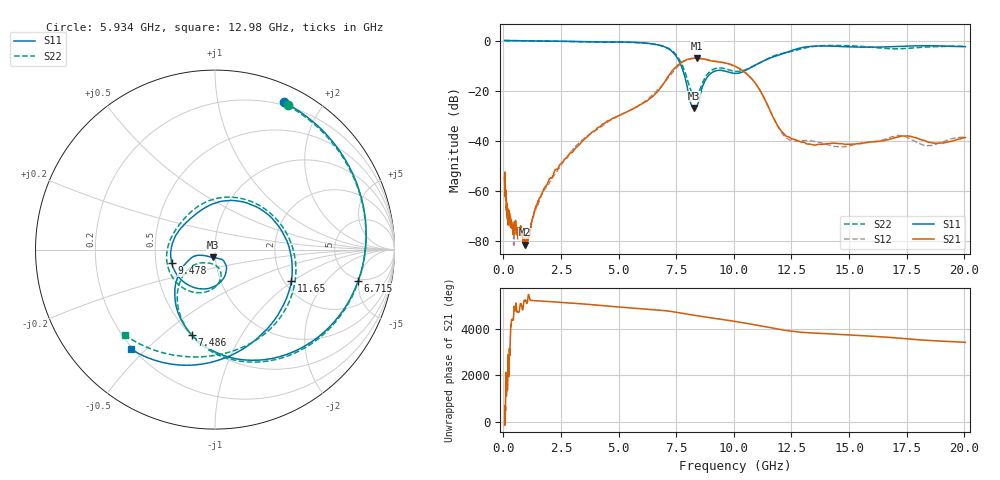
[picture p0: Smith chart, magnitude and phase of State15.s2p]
# Hz S DB R 50
!freq MagS11 AngS11 MagS21 AngS21 MagS12 AngS12 MagS22 AngS22
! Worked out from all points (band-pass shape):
!   1601 points, 50 MHz to 20.05 GHz, reference 50 ohm
!   highest |S21| = -7.06 dB at 8.407 GHz (marker M1); lowest = -81.5 dB at 946.5 MHz (marker M2)
!   |S21| within 3 dB of the highest: 7.537 GHz to 10 GHz (2.465 GHz wide, 28.1 % of centre)
!   lowest |S11| = -26.9 dB at 8.282 GHz (marker M3), VSWR 1.09, Z = 48.9 - j4.31 ohm
!   |S11| at or under -10 dB: 7.711 GHz to 10.89 GHz (3.181 GHz wide, 34.2 % of centre)
!   |S22| runs from -21.9 to 0.0 dB; largest |S21 - S12| = 0.025
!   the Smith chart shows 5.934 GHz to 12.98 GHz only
!   S11 on the Smith chart (normalised r, x): 5.934 GHz: 0.17, +1.55; 6.715 GHz: 4.71, -4.90; 7.486 GHz: 0.50, -0.64; 9.478 GHz: 0.61, -0.10; 11.65 GHz: 2.18, -0.98; 12.98 GHz: 0.19, -0.45
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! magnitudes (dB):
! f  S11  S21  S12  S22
! 50 MHz  0.0  -54.7  -54.1  0.0
! 135.9 MHz  0.0  -65.4  -66.6  0.0
! 195.5 MHz  0.0  -71.6  -73.0  0.0
! 369.6 MHz  0.0  -75.0  -73.4  0.0
! 450.8 MHz  0.0  -76.2  -81.7  0.0
! 496.9 MHz  -0.1  -73.6  -73.2  -0.1
! 946.5 MHz  -0.1  -81.5  -80.4  -0.1
! 1.005 GHz  -0.1  -79.5  -79.5  -0.1
! 2.722 GHz  -0.3  -47.0  -46.9  -0.4
! 5.934 GHz  -0.9  -25.6  -25.6  -0.9
! 6.715 GHz  -1.8  -20.1  -19.5  -1.8
! 7.402 GHz  -5.2  -11.4  -12.1  -4.8
! 7.486 GHz  -6.1  -10.6  -11.2  -5.6
! 8.282 GHz  -26.9  -7.1  -7.1  -21.8
! 8.407 GHz  -26.0  -7.1  -7.1  -21.5
! 8.893 GHz  -14.1  -7.9  -7.7  -13.0
! 9.478 GHz  -12.0  -8.7  -8.7  -11.0
! 10.69 GHz  -11.0  -14.4  -14.4  -10.9
! 11.65 GHz  -6.7  -29.6  -29.4  -6.5
! 12.27 GHz  -4.8  -38.2  -38.9  -4.8
! 12.98 GHz  -2.8  -40.6  -40.0  -3.2
! 20.05 GHz  -2.5  -38.7  -38.5  -2.3
